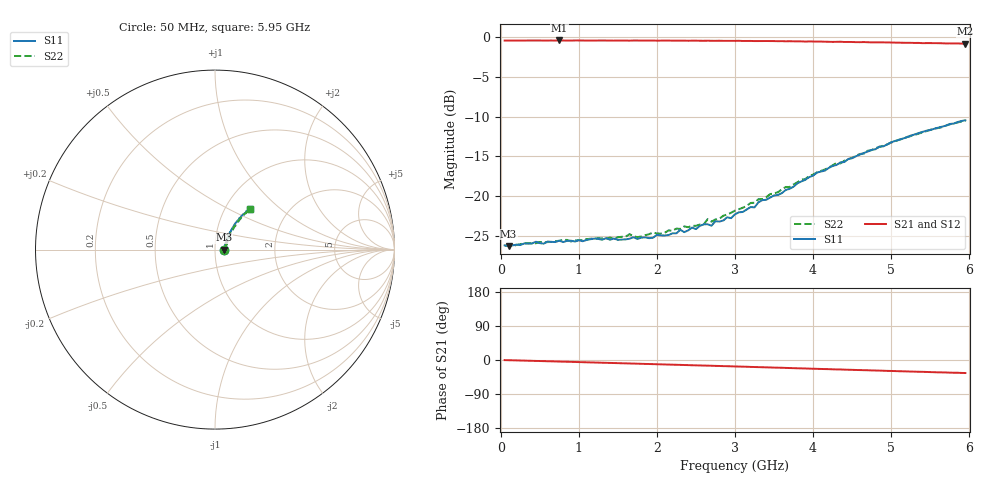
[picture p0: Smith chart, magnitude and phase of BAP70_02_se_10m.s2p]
!	Created	by	janssen	on	Thu	Dec	12	13:21:17	MET	2002
#	HZ	S	MA	R	50
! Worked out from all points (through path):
!   119 points, 50 MHz to 5.95 GHz, reference 50 ohm
!   highest |S21| = -0.41 dB at 750 MHz (marker M1); lowest = -0.8 dB at 5.95 GHz (marker M2)
!   group delay of S21, straight-line fit = 16.2 ps
!   lowest |S11| = -26.3 dB at 100 MHz (marker M3), VSWR 1.10, Z = 55.1 - j0.00637 ohm
!   |S11| at or under -10 dB: start of sweep to end of sweep
!   |S22| runs from -26.3 to -10.5 dB; largest |S21 - S12| = 0.0079
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5e7  0.04886 -0.9  0.9526 -0.3  0.951 -0.4  0.04839 -0.8
1e8  0.04846 -0.1  0.9524 -0.5  0.952 -0.6  0.04886 -0.0
7.5e8  0.05228 -0.2  0.9541 -4.1  0.9534 -4.2  0.05219 -0.7
1.05e9  0.05184 -0.4  0.9535 -5.8  0.9531 -5.8  0.05262 -1.9
1.65e9  0.05374 4.2  0.9516 -9.2  0.9529 -9.2  0.05745 3.8
1.75e9  0.05356 4.6  0.9534 -9.7  0.9526 -9.7  0.05496 5.4
2.05e9  0.05644 11.3  0.9521 -11.4  0.9517 -11.5  0.05791 9.3
2.25e9  0.05812 17.3  0.9512 -12.7  0.9522 -12.5  0.06226 14.3
2.3e9  0.06121 16.6  0.9512 -12.9  0.9517 -12.9  0.06198 16.2
2.35e9  0.05915 19.0  0.9518 -13.2  0.9516 -13.2  0.06426 16.9
2.6e9  0.06626 24.5  0.9496 -14.6  0.9517 -14.7  0.06624 21.5
2.65e9  0.06629 25.8  0.9506 -14.9  0.9499 -14.9  0.07141 22.1
2.7e9  0.06496 29.0  0.9493 -15.2  0.9493 -15.2  0.06885 25.6
2.75e9  0.06932 28.8  0.9492 -15.5  0.9491 -15.5  0.07111 26.3
2.95e9  0.07244 33.1  0.9487 -16.7  0.9492 -16.6  0.07833 31.5
3e9  0.07664 35.1  0.9485 -17.0  0.9486 -17.0  0.08082 33.4
3.25e9  0.08473 39.3  0.9456 -18.5  0.9462 -18.5  0.0906 36.7
3.35e9  0.09407 41.7  0.9461 -19.1  0.9455 -19.1  0.0955 39.2
3.6e9  0.1041 46.9  0.9448 -20.5  0.9445 -20.5  0.1101 42.2
4e9  0.1342 48.9  0.9396 -23.1  0.9393 -22.9  0.1362 47.6
5e9  0.2178 51.5  0.9261 -28.9  0.9293 -28.8  0.217 50.8
5.95e9  0.2996 48.8  0.9101 -34.4  0.9173 -34.3  0.2969 49.2
